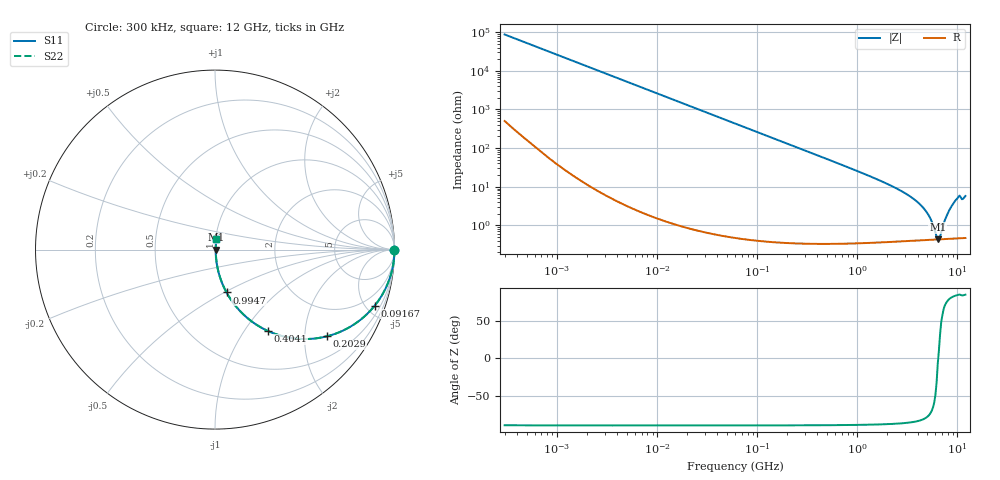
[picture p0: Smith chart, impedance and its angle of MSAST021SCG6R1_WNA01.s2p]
! MSAST021SCG6R1_WNA01  S-PARAMETER MODEL  ( General Type )
! Model Generated by TAIYO YUDEN Corporation (http://www.ty-top.com)
! Version 2.0
! TAIYO YUDEN Control No. 181101
! Copyright(c) 2015 TAIYO YUDEN CO.,LTD. All Rights Reserved.
! Product Description (link to TY-COMPAS)
! https://ds.yuden.co.jp/TYCOMPAS/or/detail?pn=MSAST021SCG6R1CWNA01&u=M
! Products Name : Multilayer Ceramic Capacitors
! Characteristics :
!  Capacitance : 6.1 pF , Rated Voltage : 25V , TCC : CG / C0G
!  Case Size : 0.25 x 0.125 / 0.0098 x 0.0049 [mm/inch] , Thickness : 0.125 / 0.0049 [mm/inch]
!  (Conditions: Temperature = 25 degC , DC Bias Current/Voltage = 0A / 0V)
! External Node Assignments :
!  1  o---| |---o  2
! GND o---------o GND
! Frequency Range : 0.3MHz  -  12000MHz  [ 401 STEP ]
# MHz S RI R 50
! Freq[MHz].  S11 Real  S11 Imag  S21 Real  S21 Imag  S12 Real  S12 Imag  S22 Real  S22 Imag
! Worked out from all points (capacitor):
!   401 points, 300 kHz to 12 GHz, reference 50 ohm
!   read as one part in series: C = 6.1 pF near 316.3 kHz
!   lowest |Z| = 438 mohm at 6.354 GHz (marker M1)
!   series resonance near 6.425 GHz, so ESL is about 100 pH
!   S11 on the Smith chart (normalised r, x): 300 kHz: open; 91.67 MHz: 1.01, -5.69; 202.9 MHz: 1.01, -2.57; 404.1 MHz: 1.01, -1.29; 994.7 MHz: 1.01, -0.51; 12 GHz: 1.01, +0.11
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0.3  1 -0.00115  7.97e-06 0.00115  7.97e-06 0.00115  1 -0.00115
1.769972  0.9999 -0.00678  5.24e-05 0.00678  5.24e-05 0.00678  0.9999 -0.00678
10.44266  0.9984 -0.04  0.00162 0.04  0.00162 0.04  0.9984 -0.04
27.82928  0.9887 -0.1054  0.0113 0.1054  0.0113 0.1054  0.9887 -0.1054
60  0.9496 -0.2183  0.0504 0.2183  0.0504 0.2183  0.9496 -0.2183
91.67136  0.8897 -0.3125  0.1103 0.3125  0.1103 0.3125  0.8897 -0.3125
202.9496  0.6222 -0.4835  0.3778 0.4835  0.3778 0.4835  0.6222 -0.4835
353.9943  0.3513 -0.4751  0.6487 0.4751  0.6487 0.4751  0.3513 -0.4751
404.1309  0.2935 -0.4528  0.7065 0.4528  0.7065 0.4528  0.2935 -0.4528
617.4538  0.1511 -0.3542  0.8489 0.3542  0.8489 0.3542  0.1511 -0.3542
994.7115  0.0643 -0.2387  0.9357 0.2387  0.9357 0.2387  0.0643 -0.2387
2088.533  0.0159 -0.1094  0.9841 0.1094  0.9841 0.1094  0.0159 -0.1094
3276.641  0.00734 -0.0581  0.9927 0.0581  0.9927 0.0581  0.00734 -0.0581
4385.161  0.00508 -0.0313  0.9949 0.0313  0.9949 0.0313  0.00508 -0.0313
5278.635  0.00446 -0.0157  0.9955 0.0157  0.9955 0.0157  0.00446 -0.0157
6188.031  0.00431 -0.00272  0.9957 0.00272  0.9957 0.00272  0.00431 -0.00272
6354.153  0.00432 -0.000568  0.9957 0.000568  0.9957 0.000568  0.00432 -0.000568
6699.894  0.00436 0.00266  0.9956 -0.00266  0.9956 -0.00266  0.00436 0.00266
7854.144  0.00476 0.0176  0.9952 -0.0176  0.9952 -0.0176  0.00476 0.0176
9207.246  0.00598 0.0379  0.994 -0.0379  0.994 -0.0379  0.00598 0.0379
10236.47  0.00757 0.0543  0.9924 -0.0543  0.9924 -0.0543  0.00757 0.0543
12000  0.00793 0.0567  0.9921 -0.0567  0.9921 -0.0567  0.00793 0.0567
